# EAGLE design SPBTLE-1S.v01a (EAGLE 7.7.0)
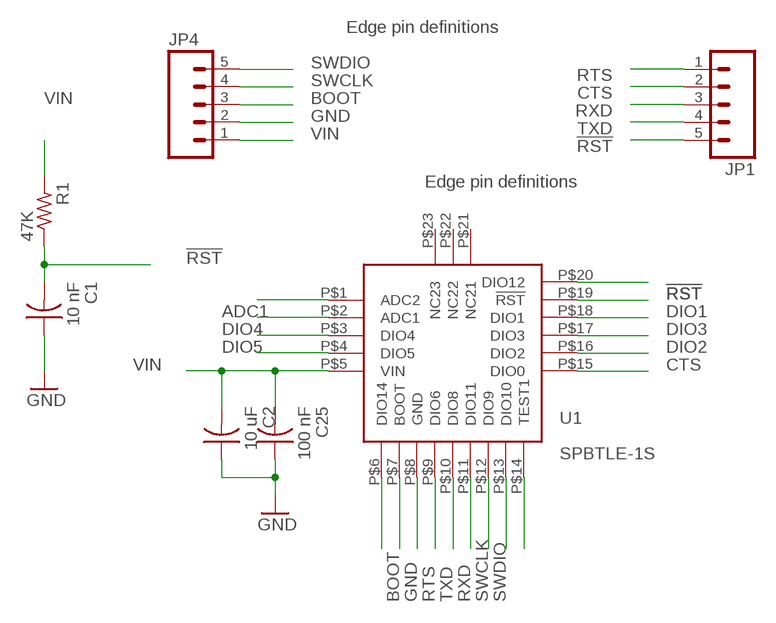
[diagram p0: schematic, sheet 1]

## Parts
C1  10 nF  C-US  [C0402_B]
C2  10 uF  C-US  [C0402_B]
C25  100 nF  C-US  [C0402_B]
JP1  M05NO_SILK  [1X05_NO_SILK]
JP4  M05NO_SILK  [1X05_NO_SILK]
R1  47K  R-US_  [R0402_B]
U1  SPBTLE-1S  [SPBTLE-1S]

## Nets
!RST: C1.2 JP1.5 R1.1 U1.P$19(!RST)
ADC1: U1.P$2(ADC1)
BOOT: JP4.3 U1.P$7(BOOT)
CTS: JP1.2 U1.P$15(DIO0)
DIO1: U1.P$18(DIO1)
DIO2: U1.P$16(DIO2)
DIO3: U1.P$17(DIO3)
DIO4: U1.P$3(DIO4)
DIO5: U1.P$4(DIO5)
GND: C1.1 C2.1 C25.1 JP4.2 U1.P$8(GND)
N$5: U1.P$20(DIO12)
N$6: U1.P$14(TEST1)
N$7: U1.P$6(DIO14)
N$11: U1.P$1(ADC2)
RTS: JP1.1 U1.P$9(DIO6)
RXD: JP1.3 U1.P$11(DIO11)
SWCLK: JP4.4 U1.P$12(DIO9)
SWDIO: JP4.5 U1.P$13(DIO10)
TXD: JP1.4 U1.P$10(DIO8)
VIN: C2.2 C25.2 JP4.1 R1.2 U1.P$5(VIN)
Unconnected: U1.P$21(NC21) U1.P$22(NC22) U1.P$23(NC23)

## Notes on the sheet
- Edge pin definitions
- Edge pin definitions

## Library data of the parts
C1 C2 C25 = Spark:C-US: Capacitor
JP1 JP4 = SparkFun-Connectors:M05: Header 5 Standard 5-pin 0.1" header. Use with straight break away headers (SKU : PRT-00116), right angle break away headers (PRT-00553), swiss pins (PRT-00743), machine pins (PRT-00117), and female headers (PRT-00115). Molex polarized connector foot print use with SKU : PRT-08230 with associated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
R1 = Spark:R-US_: 0402 Resistor
U1 = kris:SPBTLE-1S: SPBTLE-1S http://www.st.com/content/ccc/resource/technical/document/datasheet/group3/a5/eb/6a/04/8a/ad/47/9b/DM00378917/files/DM00378917.pdf/jcr:content/translations/en.DM00378917.pdf

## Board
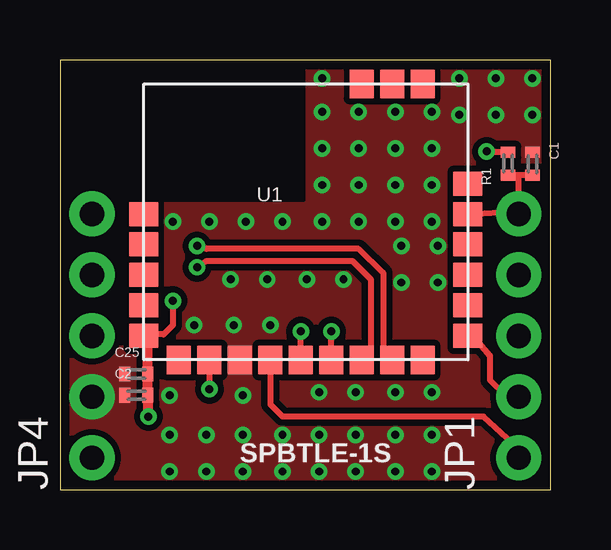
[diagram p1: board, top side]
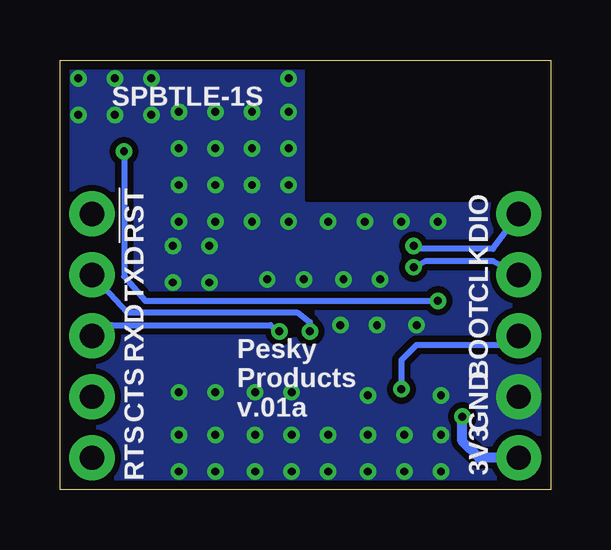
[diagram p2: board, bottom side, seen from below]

Size 20.45 x 17.91 mm. Coordinates in mm from the lower left corner, seen from the top.
Outline: 0,0 20.45,0 20.45,17.91 0,17.91 0,0
Copper layers (1*16): Top 0.0356mm / dielectric 1.5011mm / Bottom 0.0356mm
Design rules "oshpark-2layer *": minimum track width 6mil, minimum drill 13mil, track to track 6mil, track to pad 6mil, pad to pad 6mil, via to via 6mil, smd to smd 6mil, copper to edge 15mil, drill to drill 6mil, minimum pad ring 7mil, minimum via ring 7mil, stop-mask expansion 2.5mil, vias tented up to drill 20mil, thermal gap 10mil

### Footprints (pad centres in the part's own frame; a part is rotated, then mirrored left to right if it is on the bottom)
C0402_B = smd 0.457 x 0.61: 1 -0.483,0; 2 0.483,0
1X05_NO_SILK = drill 1.016 pad 1.88: 1 0,0; 2 2.54,0; 3 5.08,0; 4 7.62,0; 5 10.16,0
R0402_B = smd 0.457 x 0.61: 1 -0.483,0; 2 0.483,0
SPBTLE-1S = smd 1.2 x 1: P$1 0,6.08; P$2 0,4.81; P$3 0,3.54; P$4 0,2.27; P$5 0,1; P$15 13.5,1; P$16 13.5,2.27; P$17 13.5,3.54; P$18 13.5,4.81; P$19 13.5,6.08; P$20 13.5,7.35 | smd 1 x 1.2: P$6 1.46,0; P$7 2.73,0; P$8 4,0; P$9 5.27,0; P$10 6.54,0; P$11 7.81,0; P$12 9.08,0; P$13 10.35,0; P$14 11.62,0; P$21 11.62,11.5; P$22 10.35,11.5; P$23 9.08,11.5

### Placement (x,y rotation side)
C1  19.68,13.59 270 top
C2  3.17,3.94 0 top
C25  3.17,4.83 0 top
JP1  19.11,1.33 90 top
JP4  1.33,1.33 90 top
R1  18.67,13.59 90 top
U1  3.49,5.41 0 top

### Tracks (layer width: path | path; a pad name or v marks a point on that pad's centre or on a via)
!RST
  Top 0.254: U1.P$19 19.01,11.6 JP1.5 19.11,13.04 19.18,13.11 | C1.2 19.18,13.11 | 19.18,13.11 R1.1
BOOT  (via drill 0.33)
  Top 0.254: U1.P$7 6.22,5.08 v6.22,4.19
  Bottom 0.254: v6.22,4.19 6.22,5.4 5.59,6.03 1.71,6.03 JP4.3 | v6.22,4.19
CTS
  Top 0.254: U1.P$15 17.22,6.4 17.91,5.59 17.91,4.57 18.54,3.94 19.05,3.94 JP1.2
GND  (via drill 0.33)
  other vias: 4.7,11.18 6.22,11.18 7.75,11.18 9.27,11.18 10.92,11.18 12.45,11.18 13.97,11.18 15.49,11.18 10.92,12.7 12.45,12.7 13.97,12.7 15.49,12.7 10.92,15.75 12.45,15.75 13.97,15.75 15.49,15.75 10.92,14.22 12.45,14.22 13.97,14.22 15.49,14.22 4.57,0.76 6.1,0.76 7.62,0.76 4.57,2.29 6.1,2.29 7.62,2.29 9.27,0.76 10.79,0.76 12.32,0.76 9.27,2.29 10.79,2.29 12.32,2.29 13.97,0.76 15.49,0.76 13.97,2.29 15.49,2.29 7.62,3.94 10.79,4.06 12.32,4.06 13.97,4.06 15.49,4.06 5.59,6.86 7.24,6.86 8.76,6.86 14.22,8.64 15.75,8.64 14.22,10.16 15.75,10.16 7.11,8.76 8.64,8.76 10.29,8.76 11.81,8.76 16.64,15.62 18.16,15.62 19.68,15.62 16.64,17.14 18.16,17.14 19.68,17.14 4.57,3.94 10.92,17.14
  pour Bottom (isolate 0.254, no thermals): 0,17.91 20.45,17.91 20.45,0 0,0
  pour Top (isolate 0.254, no thermals): 0,17.91 20.45,17.91 20.45,0 0,0
N$1
  cutout Bottom (no thermals): 0,17.91 10.16,17.91 10.16,12.06 0,12.06
  cutout Top (no thermals): 0,17.91 10.16,17.91 10.16,12.06 0,12.06
RTS
  Top 0.254: U1.P$9 8.76,4.32 8.76,3.56 9.27,3.05 17.65,3.05 19.11,1.71 JP1.1
RXD  (via drill 0.33)
  Top 0.254: U1.P$11 11.3,6.73 v11.3,6.6
  Bottom 0.254: JP1.3 18.86,6.41 18.29,6.86 11.68,6.86 v11.3,6.6
SWCLK  (via drill 0.33)
  Top 0.254: v5.71,9.27 6.1,9.53 12.19,9.53 12.95,8.76 12.95,5.66 U1.P$12
  Bottom 0.254: JP4.4 2.41,9.53 5.21,9.53 v5.71,9.27
SWDIO  (via drill 0.33)
  Top 0.254: v5.71,10.16 6.1,10.03 12.45,10.03 13.46,9.05 13.46,5.92 U1.P$13
  Bottom 0.254: JP4.5 2.41,10.03 5.59,10.03 v5.71,10.16
TXD  (via drill 0.33)
  Top 0.254: U1.P$10 v10.03,6.6 | v10.03,6.6
  Bottom 0.254: v10.03,6.6 10.03,6.99 10.54,7.37 17.65,7.37 JP1.4
VIN  (via drill 0.33)
  Top 0.254: R1.2 17.93,14.07 v17.78,14.1 | v4.7,7.87 4.7,6.86 4.32,6.48 3.57,6.48 U1.P$5
  Top 0.406: U1.P$5 3.66,6.25 C25.2 C2.2 3.66,3.2 v3.68,3.05
  Bottom 0.254: v17.78,14.1 17.78,8.89 16.89,7.87 v4.7,7.87
  Bottom 0.406: JP4.1 2.98,1.33 3.68,2.03 v3.68,3.05

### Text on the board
tPlace: SPBTLE-1S
bPlace: SPBTLE-1S | !RST | DIO | CLK | TXD | BOOT | RXD | GND | CTS | 3V3 | Pesky / Products / v.01a | RTS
